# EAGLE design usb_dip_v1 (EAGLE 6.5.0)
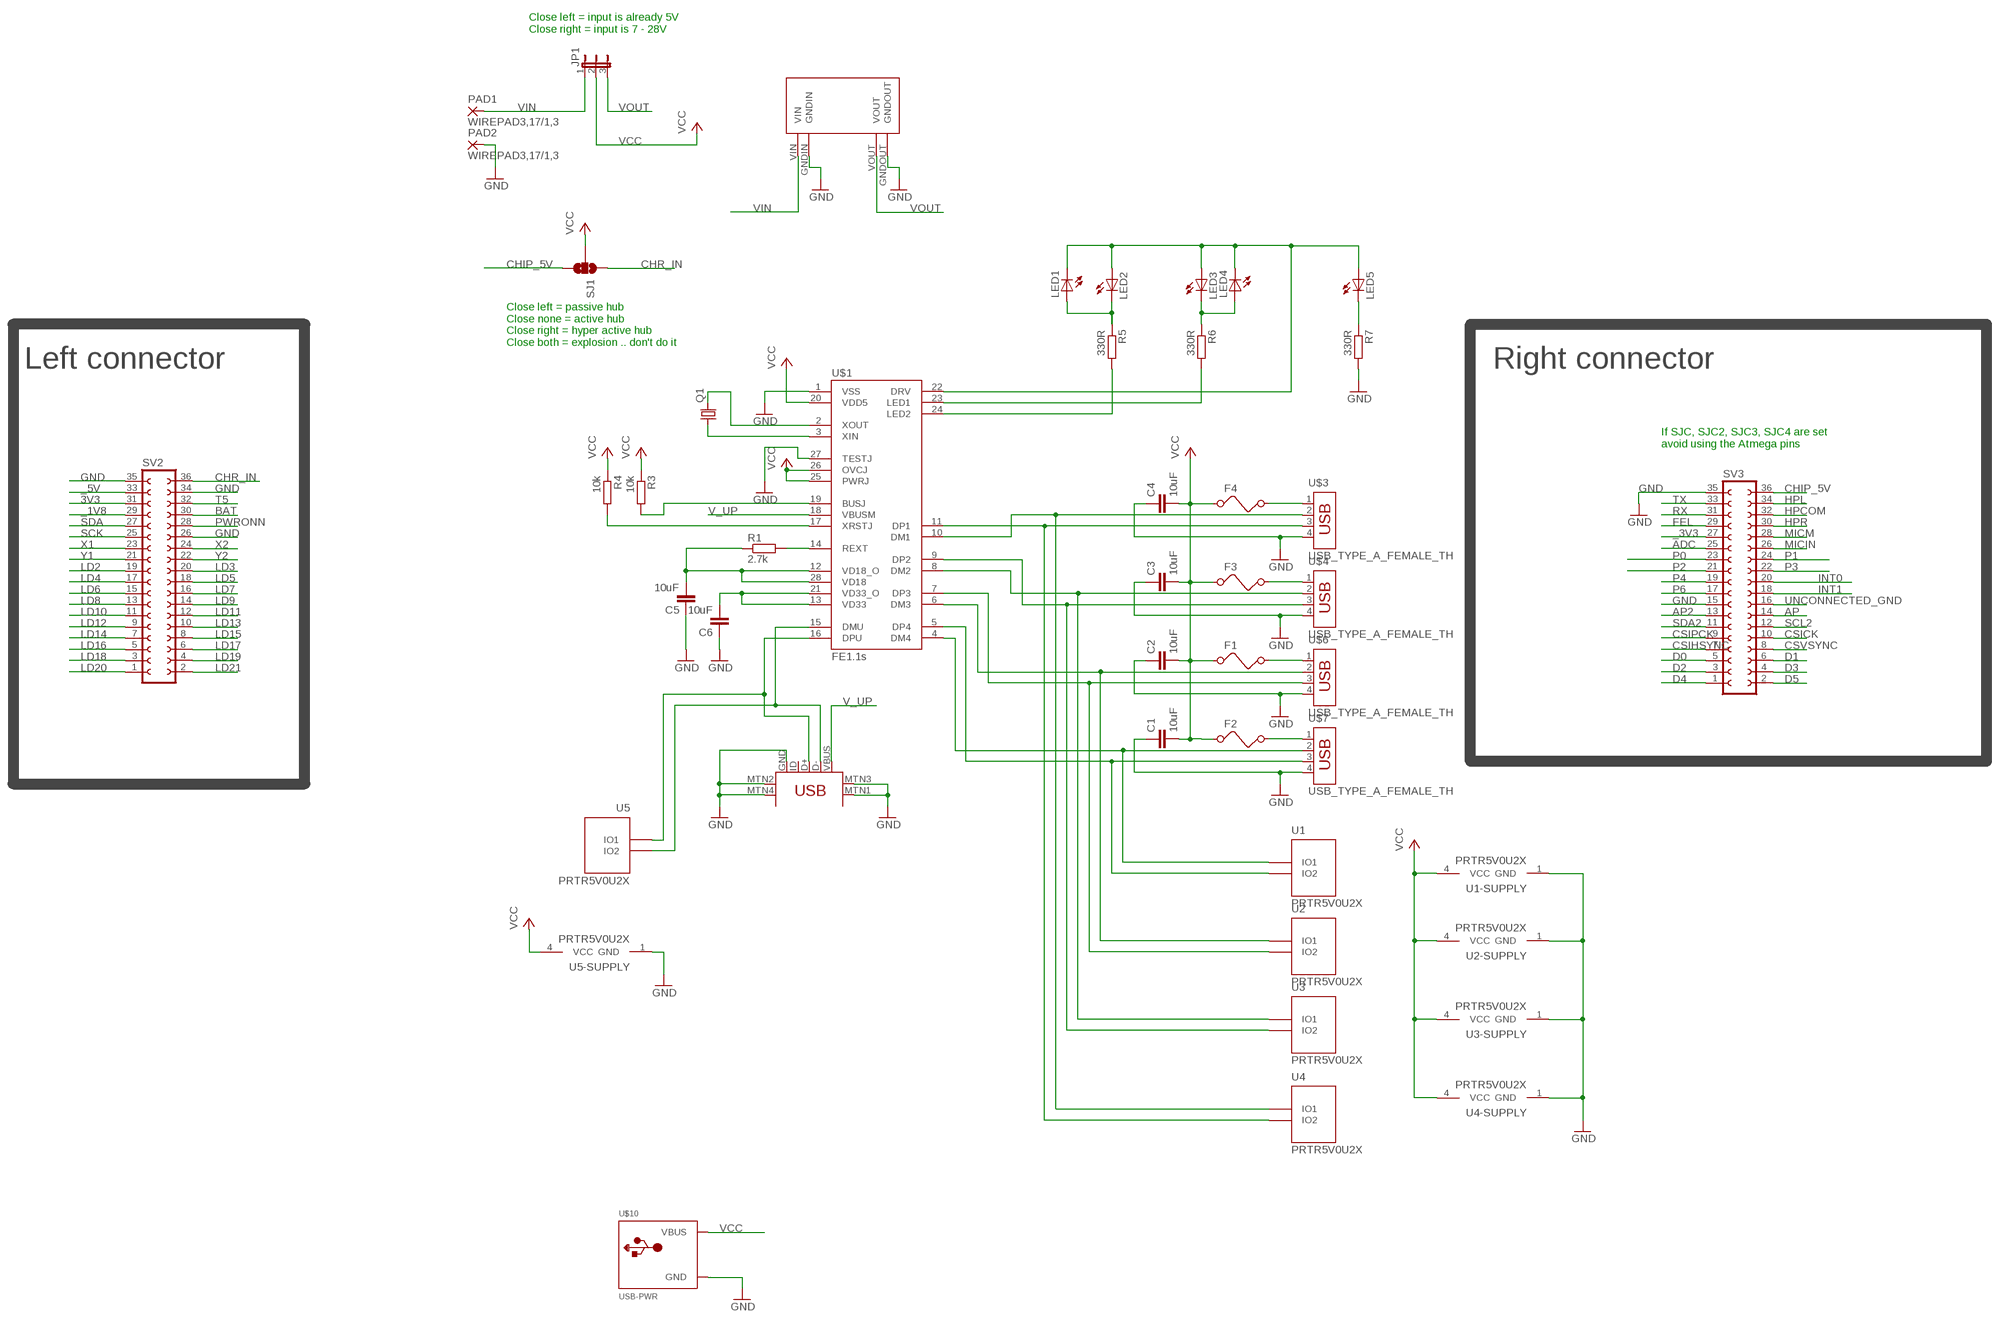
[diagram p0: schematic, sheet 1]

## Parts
C1  10uF  C-EUC1210  [C1210]
C2  10uF  C-EUC1210  [C1210]
C3  10uF  C-EUC1210  [C1210]
C4  10uF  C-EUC1210  [C1210]
C5  10uF  C-EUC1210  [C1210]
C6  10uF  C-EUC1210  [C1210]
F1  FUSED  [1210]
F2  FUSED  [1210]
F3  FUSED  [1210]
F4  FUSED  [1210]
JP1  JP2E  [JP2]
LED1  LEDCHIP-LED0805  [CHIP-LED0805]
LED2  LEDCHIP-LED0805  [CHIP-LED0805]
LED3  LEDCHIP-LED0805  [CHIP-LED0805]
LED4  LEDCHIP-LED0805  [CHIP-LED0805]
LED5  LEDCHIP-LED0805  [CHIP-LED0805]
PAD1  WIREPAD3,17/1,3  [3,17/1,3]
PAD2  WIREPAD3,17/1,3  [3,17/1,3]
Q1  CRYSTALSM49  [SM49]
R1  2.7k  R-EU_R0805  [R0805]
R3  10k  R-EU_R0805  [R0805]
R4  10k  R-EU_R0805  [R0805]
R5  330R  R-EU_R0805  [R0805]
R6  330R  R-EU_R0805  [R0805]
R7  330R  R-EU_R0805  [R0805]
SJ1  SOLDERJUMPER_2WAYT  [SJ_2]
SV2  FE18-2  [FE18-2]
SV3  FE18-2  [FE18-2]
U1  PRTR5V0U2X  [SOT-143B]
U2  PRTR5V0U2X  [SOT-143B]
U3  PRTR5V0U2X  [SOT-143B]
U4  PRTR5V0U2X  [SOT-143B]
U5  PRTR5V0U2X  [SOT-143B]
U$1  FE1.1S  [FE1.1S_SSOP-28]
U$3  USB_TYPE_A_FEMALE_TH  [USB_TYPE_A_FEMALE_TH]
U$4  USB_TYPE_A_FEMALE_TH  [USB_TYPE_A_FEMALE_TH]
U$6  USB_TYPE_A_FEMALE_TH  [USB_TYPE_A_FEMALE_TH]
U$7  USB_TYPE_A_FEMALE_TH  [USB_TYPE_A_FEMALE_TH]
U$8  USB-MINIB-5PIN  [USB-MINIB]
U$9  MP1584EN  [MP1584EN]
U$10  USB-PWR  [USB-MINIB-THM-MOLEX-PWRONLY]

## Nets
3V3: SV2.31
_1V8: SV2.29
_3V3: SV3.27
_5V: SV2.33
ADC: SV3.25
AP: SV3.14
AP2: SV3.13
BAT: SV2.30
CHIP_5V: SJ1.3 SV3.36
CHR_IN: SJ1.1 SV2.36
CSICK: SV3.10
CSIHSYNC: SV3.7
CSIPCK: SV3.9
CSVSYNC: SV3.8
D0: SV3.5
D1: SV3.6
D2: SV3.3
D3: SV3.4
D4: SV3.1
D5: SV3.2
DM1: U4.2(IO1) U$1.10(DM1) U$3.2
DM2: U3.2(IO1) U$1.8(DM2) U$4.2
DM3: U2.2(IO1) U$1.6(DM3) U$6.2
DM4: U1.2(IO1) U$1.4(DM4) U$7.2
DMU: U5.3(IO2) U$1.15(DMU) U$8.D-
DP1: U4.3(IO2) U$1.11(DP1) U$3.3
DP2: U3.3(IO2) U$1.9(DP2) U$4.3
DP3: U2.3(IO2) U$1.7(DP3) U$6.3
DP4: U1.3(IO2) U$1.5(DP4) U$7.3
DPU: U5.2(IO1) U$1.16(DPU) U$8.D+
FEL: SV3.29
GND: C1.1 C2.1 C3.1 C4.1 C5.1 C6.1 PAD2.1(P) R7.2 SV2.26 SV2.34 SV2.35 SV3.15 SV3.35 U1.1(GND) U2.1(GND) U3.1(GND) U4.1(GND) U5.1(GND) U$1.1(VSS) U$1.27(TESTJ) U$3.4 U$4.4 U$6.4 U$7.4 U$8.GND U$8.MTN1(MTN2) U$8.MTN2(MTN3) U$8.MTN3(MTN1) U$8.MTN4 U$9.GNDIN U$9.GNDOUT U$10.GND
HPCOM: SV3.32
HPL: SV3.34
HPR: SV3.30
INT0: SV3.20
INT1: SV3.18
LD2: SV2.19
LD3: SV2.20
LD4: SV2.17
LD5: SV2.18
LD6: SV2.15
LD7: SV2.16
LD8: SV2.13
LD9: SV2.14
LD10: SV2.11
LD11: SV2.12
LD12: SV2.9
LD13: SV2.10
LD14: SV2.7
LD15: SV2.8
LD16: SV2.5
LD17: SV2.6
LD18: SV2.3
LD19: SV2.4
LD20: SV2.1
LD21: SV2.2
MICIN: SV3.26
MICM: SV3.28
N$9: F2.2 U$7.1
N$10: F1.2 U$6.1
N$11: F3.2 U$4.1
N$12: F4.2 U$3.1
N$14: R5.2 U$1.24(LED2)
N$15: R6.2 U$1.23(LED1)
N$17: C6.2 U$1.13(VD33) U$1.21(VD33_O)
N$18: C5.2 R1.1 U$1.12(VD18_O) U$1.28(VD18)
N$22: R1.2 U$1.14(REXT)
N$24: R4.2 U$1.17(XRSTJ)
N$25: R3.2 U$1.19(BUSJ)
N$27: Q1.2 U$1.2(XOUT)
N$28: Q1.1 U$1.3(XIN)
N$29: LED5.C R7.1
N$30: LED3.C LED4.A R6.1
N$31: LED1.A LED2.C R5.1
N$32: LED1.C LED2.A LED3.A LED4.C LED5.A U$1.22(DRV)
P0: SV3.23
P1: SV3.24
P2: SV3.21
P3: SV3.22
P4: SV3.19
P6: SV3.17
PWRONN: SV2.28
RX: SV3.31
SCK: SV2.25
SCL2: SV3.12
SDA: SV2.27
SDA2: SV3.11
T5: SV2.32
TX: SV3.33
UNCONNECTED_GND: SV3.16
V_UP: U$1.18(VBUSM) U$8.VBUS
VCC: C1.2 C2.2 C3.2 C4.2 F1.1 F2.1 F3.1 F4.1 JP1.2 R3.1 R4.1 SJ1.2 U1.4(VCC) U2.4(VCC) U3.4(VCC) U4.4(VCC) U5.4(VCC) U$1.20(VDD5) U$1.25(PWRJ) U$1.26(OVCJ) U$10.VBUS
VIN: JP1.1 PAD1.1(P) U$9.VIN
VOUT: JP1.3 U$9.VOUT
X1: SV2.23
X2: SV2.24
Y1: SV2.21
Y2: SV2.22
Unconnected: U$8.ID

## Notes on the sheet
- Close left = input is already 5V
  Close right = input is 7 - 28V
- Close left = passive hub
  Close none = active hub
  Close right = hyper active hub
  Close both = explosion .. don't do it
- Left connector | Right connector
- If SJC, SJC2, SJC3, SJC4 are set 
  avoid using the Atmega pins

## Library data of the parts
C1-C6 = rcl:C-EU: CAPACITOR, European symbol
F1-F4 = m-pad-2.1:FUSE: Fuse's in various packages
JP1 = jumper:JP2E: JUMPER
LED1-LED5 = led:LED: LED
PAD1 PAD2 = wirepad:WIREPAD: Wire PAD connect wire on PCB
Q1 = adafruit:CRYSTAL: CRYSTAL; OC_FARNELL: unknown; OC_NEWARK: unknown
R1 R3-R7 = rcl:R-EU_: RESISTOR, European symbol
SJ1 = SparkFun-Retired:SOLDERJUMPER_2WAY: Solder Jumper 2 way solder jumper
SV2 SV3 = con-lsta:FE18-2: FEMALE HEADER; OC_FARNELL: unknown; OC_NEWARK: unknown
U1-U5 = Volks73-NXPSemiconductors:PRTR5V0U2X?: I2C-Bus EDS Protection Ulta low capacitance double rail-to-rail ESD protection diode Documentation Datasheet General Description Ultra low capacitance rail-to-rail ElectroStatic Discharge (ESD) protection diode in a small SOT143B Surface-Mounted Device (SMD) plastic package designed to protect two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; APPLICATIONS: General Purpose; BIDIRECTIONAL_CHANNELS: 2; CAPACITANCE: 1pF @ 1MHz; CURRENT_PEAK_PULSE: -; DESCRIPTION: TVS DIODE 5.5VWM SOT143B; DOCUMENTATION_LINK: <a href="http://www.nxp.com/documents/data_sheet/PRTR5V0U2X.pdf">Datasheet</a>; DOCUMENTATION_URL: http://www.nxp.com/documents/data_sheet/PRTR5V0U2X.pdf; MANUFACTURER: NXP Semiconductors; MOUNTING_TYPE: Surface Mount; OPERATING_TEMPERATURE: -40C ~ 85C; PART_NUMBER: PRTR5V0U2X,215; POWER-PEAK_PULSE: -; POWER_LINE_PROTECTION: Yes; SUPPLIER_ITEM_LINK: <a href="http://www.digikey.com/product-detail/en/PRTR5V0U2X,215/568-4140-1-ND/1589981">Details</a>; SUPPLIER_ITEM_NUMBER: 568-4140-1-ND; SUPPLIER_ITEM_URL: http://www.digikey.com/product-detail/en/PRTR5V0U2X,215/568-4140-1-ND/1589981; SUPPLIER_LINK: <a href="http://www.digikey.com">Home Page</a>; SUPPLIER_NAME: Digi-Key; SUPPLIER_URL: http://www.digikey.com; TYPE: Steering (Rail to Rail); UNIDIRECTIONAL_CHANNELS: -; VOLTAGE_BREAKDOWN: 6V; VOLTAGE_CLAMPING: -; VOLTAGE_REVERSE: 5.5V
U$1 = imcom:FE1.1S: A USB 2.0 hub IC. http://www.jfd-ic.com/Documents/FE1.1s%20Data%20Sheet%20%28Rev.%201.0%29.pdf
U$3 U$4 U$6 U$7 = imcom:USB_TYPE_A_FEMALE_TH: USB Type A Female Through Hole. http://datasheet.octopart.com/787616-1-Tyco-Electronics-datasheet-61477.pdf
U$8 = SparkFun-Connectors:USB-MINIB: Mini-USB "B" connector with 5th pin broken out. Created new symbol breaking out 5th "ID" pin in mini/micro USB connector spec. See: http://en.wikipedia.org/wiki/Mini_usb#Cables. Uses same footprint as 4-pin symbol. Also added pins to connect to mounting / shield pads if required (probably not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
U$9 = power_supply:MP1584EN
U$10 = adafruit:USB-PWR

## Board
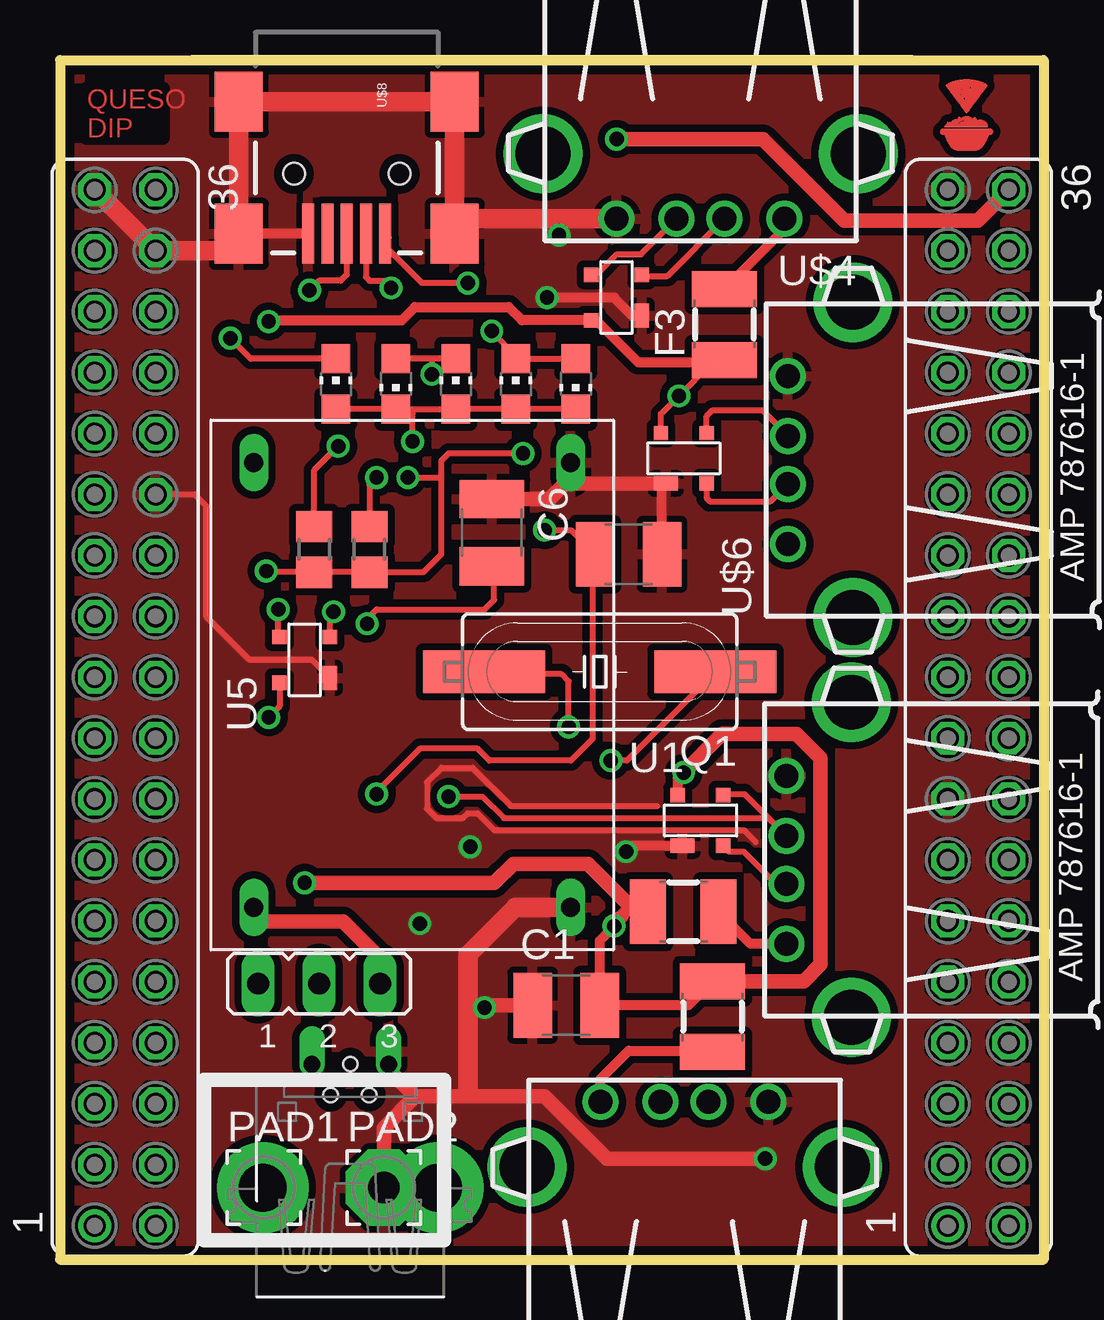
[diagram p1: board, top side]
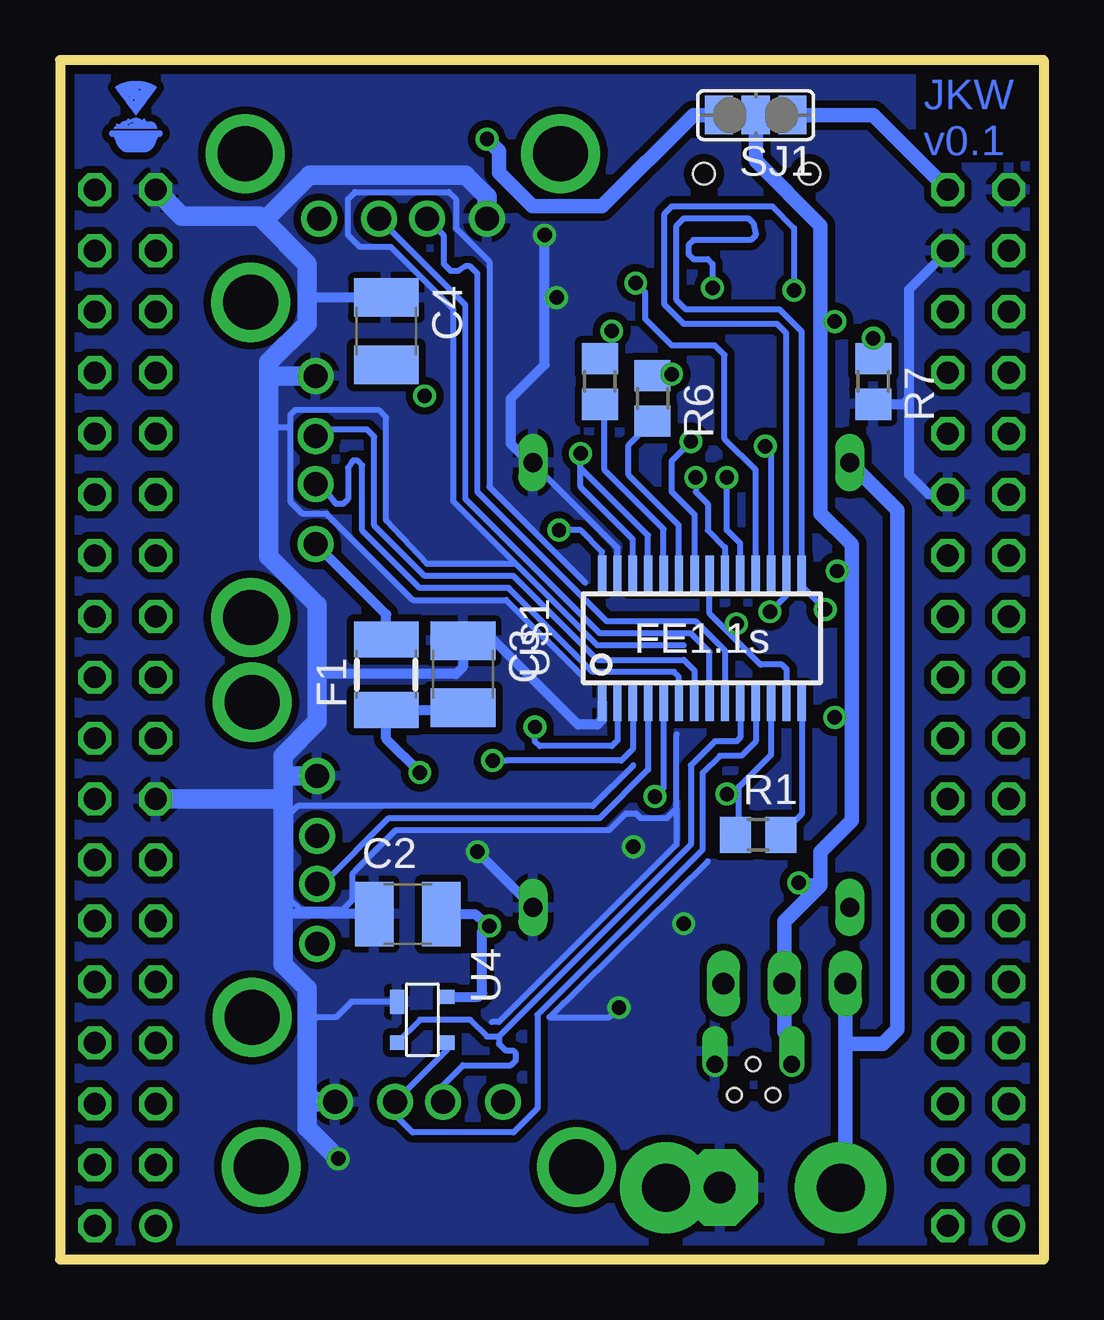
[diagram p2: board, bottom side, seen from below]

Size 41 x 50 mm. Coordinates in mm from the lower left corner, seen from the top.
Outline: 0,50 41,50 41,0 0,0 0,50
Copper layers (1*16): Top 0.0356mm / dielectric 1.5011mm / Bottom 0.0356mm
Design rules "LaenPCBOrder": minimum track width 6mil, minimum drill 13mil, track to track 6mil, track to pad 6mil, pad to pad 6mil, via to via 6mil, smd to smd 6mil, copper to edge 15mil, drill to drill 6mil, minimum pad ring 7mil, minimum via ring 7mil, stop-mask expansion 3mil, vias tented up to drill 0mil, thermal gap 10mil

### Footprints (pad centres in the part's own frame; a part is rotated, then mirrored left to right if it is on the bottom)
C1210 = smd 1.6 x 2.7: 1 -1.4,0; 2 1.4,0
1210 = smd 1.5 x 2.7: 1 -1.5,0; 2 1.45,0
JP2 = drill 0.914 long: 1 -2.54,0; 2 0,0; 3 2.54,0
CHIP-LED0805 = smd 1.2 x 1.2: A 0,-1.05; C 0,1.05
3,17/1,3 = drill 1.321 pad 3.175 octagon: 1 0,0
SM49 = smd 5.08 x 1.778: 1 -4.826,0; 2 4.826,0
R0805 = smd 1.3 x 1.5: 1 -0.95,0; 2 0.95,0
SJ_2 = smd 1.168 x 1.6: 1 -1.524,0; 2 0,0; 3 1.524,0
FE18-2 = drill 0.914: 1 -21.59,1.27 | drill 0.914 octagon: 2 -21.59,-1.27; 3 -19.05,1.27; 4 -19.05,-1.27; 5 -16.51,1.27; 6 -16.51,-1.27; 7 -13.97,1.27; 8 -13.97,-1.27; 9 -11.43,1.27; 10 -11.43,-1.27; 11 -8.89,1.27; 12 -8.89,-1.27; 13 -6.35,1.27; 14 -6.35,-1.27; 15 -3.81,1.27; 16 -3.81,-1.27; 17 -1.27,1.27; 18 -1.27,-1.27; 19 1.27,1.27; 20 1.27,-1.27; 21 3.81,1.27; 22 3.81,-1.27; 23 6.35,1.27; 24 6.35,-1.27; 25 8.89,1.27; 26 8.89,-1.27; 27 11.43,1.27; 28 11.43,-1.27; 29 13.97,1.27; 30 13.97,-1.27; 31 16.51,1.27; 32 16.51,-1.27; 33 19.05,1.27; 34 19.05,-1.27; 35 21.59,1.27; 36 21.59,-1.27
SOT-143B = smd 1 x 0.6: 1 -0.75,-1.05 | smd 0.6 x 0.6: 2 0.95,-1.05; 3 0.95,1.05; 4 -0.95,1.05
FE1.1S_SSOP-28 = smd 0.35 x 1.5: 1 -4.16,-2.7; 2 -3.52,-2.7; 3 -2.88,-2.7; 4 -2.24,-2.7; 5 -1.6,-2.7; 6 -0.96,-2.7; 7 -0.32,-2.7; 8 0.32,-2.7; 9 0.96,-2.7; 10 1.6,-2.7; 11 2.24,-2.7; 12 2.88,-2.7; 13 3.52,-2.7; 14 4.16,-2.7; 15 4.16,2.7; 16 3.52,2.7; 17 2.88,2.7; 18 2.24,2.7; 19 1.6,2.7; 20 0.96,2.7; 21 0.32,2.7; 22 -0.3,2.7; 23 -0.96,2.7; 24 -1.6,2.7; 25 -2.24,2.7; 26 -2.88,2.7; 27 -3.52,2.7; 28 -4.16,2.7
USB_TYPE_A_FEMALE_TH = drill 1: 1 -3.5,5.37; 2 -1,5.37; 3 1,5.37; 4 3.5,5.37 | drill 2.286: P$1 -6.57,2.66; P$2 6.57,2.66
USB-MINIB = smd 2.5 x 0.5: D+ 2.5,0; D- 2.5,0.8; GND 2.5,-1.6; ID 2.5,-0.8; VBUS 2.5,1.6 | smd 2.5 x 2: MTN1 -3,4.5; MTN2 2.5,4.5; MTN3 -3,-4.5; MTN4 2.5,-4.5 | hole 0.9: 0,2.2; 0,-2.2
MP1584EN = drill 0.8 long: GNDIN 1.778,14.986; GNDOUT 20.32,14.986; VIN 1.778,1.778; VOUT 20.32,1.778
USB-MINIB-THM-MOLEX-PWRONLY = drill 0.7 offset: GND 1.6,4.64; VBUS -1.6,4.64 | drill 2 pad 3.81: GND1 -3.65,-0.51; GND4 3.65,-0.51 | hole 0.6: 0,4.648; 0.787,3.353; -0.813,3.353

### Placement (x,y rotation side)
C1  21.1,10.6 0 top
C2  26.5,14.4 0 bottom
C3  24.2,24.4 270 bottom
C4  27.4,38.7 270 bottom
C5  23.7,29.4 180 top
C6  18,30.3 270 top
F1  27.4,24.4 90 bottom
F2  26,14.5 0 top
F3  27.7,39 90 top
F4  27.2,10.1 270 top
JP1  10.8,11.5 0 top
LED1  21.5,36.5 180 top
LED2  19,36.5 0 top
LED3  16.5,36.5 0 top
LED4  14,36.5 180 top
LED5  11.5,36.5 0 top
PAD1  8.5,3 0 top
PAD2  13.5,3 0 top
Q1  22.5,24.5 180 top
R1  11.9,17.7 0 bottom
R3  12.9,29.6 90 top
R4  10.6,29.6 90 top
R5  18.5,36.6 270 bottom
R6  16.3,35.9 270 bottom
R7  7.1,36.6 270 bottom
SJ1  12,47.7 180 bottom
SV2  2.72,23 90 top
SV3  38.28,23 90 top
U1  26.7,18.3 0 top
U2  26,33.4 0 top
U3  23.2,40.1 90 top
U4  25.9,10 270 bottom
U5  10.2,25 90 top
U$1  14.24,25.9 0 bottom
U$2  LOGO  [LOGO]  36.54,46.02 0 top
U$3  26.04,1.2 0 top
U$4  26.71,48.75 180 top
U$5  LOGO  [LOGO]  39.09,46.1 0 bottom
U$6  35.71,33.33 90 top
U$7  35.65,16.66 90 top
U$8  11.95,45.25 270 top
U$9  6.3,35 270 top
U$10  12.1,3.5 0 top

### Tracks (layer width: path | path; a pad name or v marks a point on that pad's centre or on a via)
CHIP_5V  (via drill 0.6)
  Top 0.61: v23.2,46.7 29.3,46.7 32.7,43.3 38.26,43.3 SV3.36
  Bottom 0.61: v23.2,46.7 22.7,46.2 22.7,45.3 21.3,43.9 18.4,43.9 14.6,47.7 SJ1.3
CHR_IN
  Bottom 0.61: 4.2,44.8 SV2.36 7.1,47.7 SJ1.1
DM1
  Bottom 0.254: 25.04,6.96 U$3.2 25.04,7.26 24.2,8.1 22.2,8.1 22,8.3 22,8.6 22.1,8.7 22.4,8.7 22.7,9 22.7,9.3 | U4.2 26,10 23.9,10 23.2,9.3 22.7,9.3 | U$1.10 12.64,21.76 12.8,21.6 13.7,21.6 14.7,20.6 14.7,17.3 22.7,9.3
DM2
  Top 0.254: 27.71,43.31 U$4.2 25.33,41 24.3,41 U3.2
  Bottom 0.254: U$1.8 13.92,25.32 14.7,26.1 18.5,26.1 24.1,31.7 24.1,39.77 U$4.2
DM3
  Top 0.254: 26.9,32.3 U2.2 26.95,31.75 27.1,31.6 29.61,31.6 U$6.2
  Bottom 0.254: U$1.6 15.2,24.3 15.4,24.5 18.8,24.5 22.3,28 26.01,28 28.4,30.39 28.4,33.1 28.6,33.3 28.8,33.3 29,33 29,31.7 29.2,31.5 29.5,31.5 30.13,32.33 U$6.2
DM4
  Top 0.254: U$7.2 29.84,15.66 28.5,17 27.9,17 U1.2
  Bottom 0.254: U$1.4 16.48,20.42 18.5,18.4 27.3,18.4 30.04,15.66 U$7.2
DMU  (via drill 0.6)
  Top 0.254: U$8.D- 12.75,40.95 12.9,40.8 13.5,40.8 v13.8,40.5 | U5.3 9.1,26 v9.1,27.1
  Bottom 0.254: v13.8,40.5 13.8,41.5 14,41.7 14.6,41.7 14.8,41.9 14.8,42.3 14.6,42.5 12.2,42.5 12,42.7 12.1,43.2 12.3,43.4 15,43.4 15.3,43.1 15.3,40 14.9,39.6 11,39.6 10.08,38.68 U$1.15 10.08,28.08 v9.1,27.1
DP1
  Bottom 0.254: U4.3 24.85,8.76 U$3.3 27.04,6.04 26.3,5.3 22.1,5.3 21.1,6.3 21.1,10.2 14.2,17.1 14.2,20.3 13.5,21 12.6,21 12,21.6 U$1.11
DP2
  Top 0.254: U3.3 22.1,41.1 22.4,41.1 23.2,41.9 24.23,41.9 U$4.3
  Bottom 0.254: U$1.9 13.28,25.38 14.5,26.6 18.2,26.6 23.6,32 23.6,41.1 23.9,41.4 24.1,41.4 24.4,41.2 24.7,41.2 25,41.5 25,42.67 U$4.3
DP3
  Top 0.254: U2.3 26.95,35.15 27.2,35.4 29.27,35.4 U$6.3
  Bottom 0.254: U$1.7 14.56,24.56 15,25 18.6,25 22.1,28.5 25.8,28.5 27.9,30.6 27.9,34.3 28.2,34.6 30.07,34.6 U$6.3
DP4  (via drill 0.6)
  Top 0.254: U1.3 27.7,19.4 28.54,19.4 U$7.3 | 29.34,18.6 U$7.3 | v16.2,19.3 17.6,19.3 18.5,18.4 29.54,18.4 U$7.3
  Bottom 0.254: U$1.5 15.84,19.66 v16.2,19.3
DPU  (via drill 0.6)
  Top 0.254: U$8.D+ 11.95,41.05 11.7,40.8 10.8,40.8 v10.4,40.4 | U5.2 11.25,26.85 v11.4,27
  Bottom 0.254: v10.4,40.4 10.4,43 11.3,43.9 15.5,43.9 15.8,43.6 15.8,39.8 15,39 11.1,39 10.72,38.62 U$1.16 10.7,28.58 10.7,27.7 v11.4,27
GND  (via drill 0.6)
  Top 0.254: 29,17.4 28.5,17.9 18.1,17.9 17.4,18.6 17,18.6 16.8,18.4 15.7,18.4 15.3,18.8 15.3,19.9 15.9,20.5 17.2,20.5 18.8,18.9 24.9,18.9 | U5.1 10.5,25 7.9,25 6.1,26.8 6.1,31.4 5.61,31.89 SV2.26
  Top 0.406: U$8.GND U$8.MTN4 | v20.8,42.7 20.8,43.38 | U3.1 23.85,39.35 23.1,40.1 v20.3,40.1 | U1.1 23.85,17.25 v23.6,17 | C5.1 25.1,32.2 U2.1
  Top 0.61: C6.1 20.4,31.7 21.3,32.6 | U2.1 21.55,32.35 21.3,32.6 | 21.3,32.6 21.3,33.21 U$9.GNDIN | PAD2.1 13.5,5.5 14.8,6.8 | 14.8,6.8 20.2,6.8 22.8,4.2 v29.4,4.2 | 14.8,6.8 13.7,7.9 U$10.GND | C1.1 17.1,10.6 17,10.5
  Top 0.813: U$4.4 20.8,43.38 17.08,43.38 16.85,43.15 | 16.85,43.15 U$8.MTN2 | 16.85,43.15 16.45,43.55 U$8.MTN1 U$8.MTN3 U$8.MTN4 6.75,42.05 SV2.34 SV2.35 | U$9.GNDOUT 18.98,14.68 17,12.7 17,10.5 17,7
  Bottom 0.254: U4.1 28.85,10.75 29.5,10.1 30.3,10.1 30.7,9.7 | 15,25.6 18.6,25.6 24.6,31.6 24.6,39.6 27.2,42.2 28.5,42.2 29,42.7 29,44.2 28.7,44.5 24.8,44.5 24.5,44.2 24.5,43 23.1,41.6 23.1,32.2 19.1,28.2 | 22.1,29 25.7,29 27.4,30.8 27.4,35.1 27.7,35.4 31.2,35.4 31.4,35.2 31.4,34.6 | 31.4,34.6 31.4,31.6 30.9,31.1 29.9,31.1 26.3,27.5 22.4,27.5 19.2,24.3 | 17.1,20.6 18.8,18.9 31.1,18.9 31.4,18.6 | 31.4,18.6 31.4,15 31,14.6 29.2,14.6 28.8,15 28.8,16.1 27,17.9 18.1,17.9 17.4,18.6 17,18.6 16.8,18.4 15.7,18.4 15.3,18.8 | 15.3,18.8 15.3,21.9 | 15.3,18.8 15.3,17.3 22.7,9.9 23,9.9 | 14,16.6 20.6,10.1 18.1,10.1 v17.7,10.5 | 32.3,34.7 31.5,34.7 31.4,34.6 | 31.4,18.6 31.5,18.6 31.7,18.8 | U$1.27 17.76,29.66 20.72,32.62 U$9.GNDIN
  Bottom 0.406: 30.18,23.3 30.28,23.2 | U$1.1 18.4,22.5 18.6,22.3 19.4,22.3 22.9,25.8 C3.1 24.2,24.7 24.5,24.4 30.28,24.4 | U$9.GNDIN 21.29,33.09 22.2,34 22.2,35.9 20.8,37.3 20.8,40.1 | 20.8,40.1 v20.8,42.7 | C2.1 31.7,14.4 | C4.1 30.7,40.1 | v20.3,40.1 20.8,40.1 | U$9.GNDOUT 21.3,14.09 21.3,14.7 v23.6,17 | SV2.26 4.79,31.89 5.6,32.7 5.6,35.9 | 5.6,35.9 5.6,40.44 SV2.34 | R7.2 5.85,35.65 5.6,35.9
  Bottom 0.813: 32.3,36.9 32.3,34.7 32.3,29.3 30.28,27.28 30.28,24.4 30.28,23.2 30.28,22.42 31.7,21 31.7,20.1 | 32.3,36.9 32.3,37.4 30.7,39 30.7,40.1 30.7,41.5 32.5,43.3 | 32.5,43.3 32.7,43.5 35.92,43.5 SV3.35 | 31.7,20.1 31.7,18.9 | 31.7,18.9 31.7,18.8 31.7,14.4 31.7,12.3 30.7,11.3 30.7,9.7 30.7,6.9 | 30.7,6.9 30.7,5.5 v29.4,4.2 | U$3.4 30.37,6.57 30.7,6.9 | U$7.4 31.64,20.16 31.7,20.1 | SV3.15 31.99,19.19 31.7,18.9 | U$6.4 32.23,36.83 32.3,36.9 | U$4.4 23.21,44.31 24.1,45.2 30.6,45.2 32.5,43.3
  other vias: 17.1,17.2 15,14
  pour Top (isolate 0.305, rank 2): -0.07,0.25 40.88,0.25 41.01,10.57 41.01,50.01 0,50.01 0,10.47
  pour Bottom (isolate 0.305): 0,50 41.05,50 41.05,0.25 0.02,0.25 0.02,49.92
N$9
  Top 0.406: U$7.1 28.79,13.16 F2.2
N$10
  Bottom 0.406: F1.2 27.4,26.89 U$6.1
N$11
  Top 0.406: U$4.1 30.21,42.96 F3.2
N$12
  Top 0.406: U$3.1 22.54,7.54 23.7,8.7 27.15,8.7 F4.2
N$14
  Bottom 0.254: 18.25,35.4 R5.2 18.3,35.45 18.3,32.9 15.84,30.44 U$1.24
N$15
  Bottom 0.254: U$1.23 15.2,30.6 17.3,32.7 17.3,33.95 R6.2
N$17  (via drill 0.6)
  Top 0.254: v12.8,26.5 12.8,26.7 13.2,27.1 17.7,27.1 18.1,27.5 18.1,28.8 C6.2 17.8,28.7
  Bottom 0.254: U$1.13 10.7,23.22 10.7,24.6 10.9,24.8 11.8,24.8 13.05,26.05 | 13.05,26.05 13.92,26.92 U$1.21 | v12.8,26.5 13.05,26.25 13.05,26.05
N$18  (via drill 0.6)
  Top 0.254: C5.2 22,29.4 | v20.2,30.4 21.3,30.4 C5.2 | C5.2 22.2,29.3 22.2,21.7 21.3,20.8 17.9,20.8 17.4,21.3 15,21.3 13.2,19.5 v13.2,19.4
  Bottom 0.254: U$1.12 11.36,21.04 12.7,19.7 12.7,19.4 | R1.1 12.7,17.85 12.7,19.4 | v13.2,19.4 12.7,19.4 | U$1.28 18.4,29.5 19.3,30.4 v20.2,30.4
N$22
  Bottom 0.254: U$1.14 10.08,18.57 R1.2
N$24  (via drill 0.6)
  Top 0.254: R4.2 10.6,32.9 v11.6,33.9
  Bottom 0.254: v11.6,33.9 11.36,33.66 U$1.17
N$25  (via drill 0.6)
  Top 0.254: v13.2,32.6 12.9,32.3 R3.2
  Bottom 0.254: U$1.19 12.64,29.84 13.2,30.4 v13.2,32.6
N$27  (via drill 0.6)
  Top 0.254: v21.2,22.2 21.2,24.1 20.9,24.4 17.77,24.4 Q1.2
  Bottom 0.254: U$1.2 17.76,21.64 18,21.4 21,21.4 21.2,21.6 v21.2,22.2
N$28  (via drill 0.6)
  Top 0.254: Q1.1 23.63,20.8 v22.96,20.8
  Bottom 0.254: U$1.3 17.12,21.28 17.6,20.8 22.4,20.8 v22.96,20.8
N$29  (via drill 0.6)
  Top 0.254: LED5.C 7.95,37.55 v7.1,38.4
  Bottom 0.254: v7.1,38.4 R7.1
N$30  (via drill 0.6)
  Top 0.254: LED3.C 15.5,37.55 | 15.5,37.55 LED4.A | v15.5,36.9 15.5,37.55
  Bottom 0.254: R6.1 15.55,36.85 v15.5,36.9
N$31  (via drill 0.6)
  Top 0.254: LED1.A LED2.C 19,37.6 v18,38.7
  Bottom 0.254: v18,38.7 18,38.05 R5.1
N$32  (via drill 0.6)
  Top 0.254: LED1.C LED2.A LED3.A 14.5,35.45 | 13.9,35.45 LED4.C | LED4.C LED5.A | LED4.C 14.5,35.45 | v14.7,34.1 14.7,35.25 14.5,35.45
  Bottom 0.254: U$1.22 14.54,31.04 15.5,32 15.5,33.3 v14.7,34.1
V_UP  (via drill 0.6)
  Top 0.254: v17,40.7 15.1,40.7 13.7,42.1 13.7,42.6 U$8.VBUS
  Bottom 0.254: U$1.18 12,32.9 13.3,34.2 13.3,37.7 13.7,38.1 15.5,38.1 16.6,39.2 16.6,40.3 v17,40.7
VCC  (via drill 0.6)  (1 unrouted)
  Top 0.254: v8.6,28.7 8.65,28.65 R4.1 R3.1 15.15,28.65 15.9,29.4 15.9,32.5 | F3.1 27.5,37.3 C4.2 27.1,37.3 v25.8,36 25.05,35.25 U2.4 | U5.4 9.15,23.05 v8.7,22.6 | 15.9,32.5 15.9,33.3 16.2,33.6 v19.3,33.6 | v14.5,32.6 15.8,32.6 15.9,32.5
  Top 0.406: 23.5,14.5 24,14.5 F2.1 | 23.2,14.2 23.5,14.5 | v8.7,39.1 8.75,39.15 14.25,39.15 14.8,39.7 18.7,39.7 19.25,39.15 U3.4 22.35,39.15 24.1,37.4 27.3,37.4 C4.2 | F3.1 26.5,37.5 | U1.4 25.75,20.05 v26,20.3 | F4.1 26.2,10.6 C1.2 22.5,13.3 v23.1,13.9 23.5,14.3 23.5,14.5
  Top 0.61: F4.1 31,11.6 31.7,12.3 31.7,20.9 30.7,21.9 27.6,21.9 v26,20.3 | 24,14.5 22,16.5 18.9,16.5 18.1,15.7 v10.2,15.7
  Bottom 0.254: v8.6,28.7 8,28.7 | v8.7,22.6 8,22.6 | U$1.26 17.12,30.02 19.3,32.2 v19.3,33.6 19.3,33 16.48,30.18 U$1.25 | v14.5,32.6 14.5,32 14,31.5 14,30.4 13.28,29.68 U$1.20
  Bottom 0.406: v10.2,15.7 9.4,15.7 9.3,15.6 | C2.2 23.7,14.4 v23.1,13.9 23.4,13.7 23.4,11.1 23.55,10.95 U4.4 | v8.7,39.1 9.2,39.1 9.3,39.2 | v26,20.3 27.4,21.7 F1.1 24.3,22.9 C3.2
  Bottom 0.61: SJ1.2 12,45.8 9.3,43.1 9.3,39.2 9.3,31.1 8,29.8 8,28.7 8,22.6 8,18.3 9.3,17 9.3,15.6 10.8,14.1 JP1.2 10.8,9.5 10.5,9.2 U$10.VBUS
VIN
  Bottom 0.61: U$9.VIN 6.1,31.24 6.1,9.6 6.7,9 8.26,9 | PAD1.1 8.26,3.24 8.26,9 | 8.26,9 JP1.1
VOUT
  Top 0.61: JP1.3 13.34,12.56 11.8,14.1 8.1,14.1 U$9.VOUT

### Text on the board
Top: QUESO / DIP
Bottom: JKW / v0.1
tStop: SALSA / DIP
bStop: JKW / v3.9

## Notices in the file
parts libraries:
SparkFun-Connectors: Licensing: Creative Commons ShareAlike 4.0 International - https://creativecommons.org/licenses/by-sa/4.0
m-pad-2.1: License : GNU General Public License version 2 (see bottom)
